(* Logix 5000 AddOnInstructionDefinition export Banner_Q5X_2000_Param_v4; software revision 33.00; part 2 of 3 *)
(* tags used below, declared in another part *)
   Q5X : Banner_Q5X_2000_v4;
   Port_Data : Banner_IOL_Port_v4;
   Port : DINT;
   Local_Control : DINT;
   Command_Being_Processed : BOOL;
   Update_Archive : BOOL;
   Index_Write_Inprocess : INT;
   Index_Write_Control : INT;
   Inprocess_Index : DINT;
(* Banner_Q5X_2000_Param_v4, continued *)

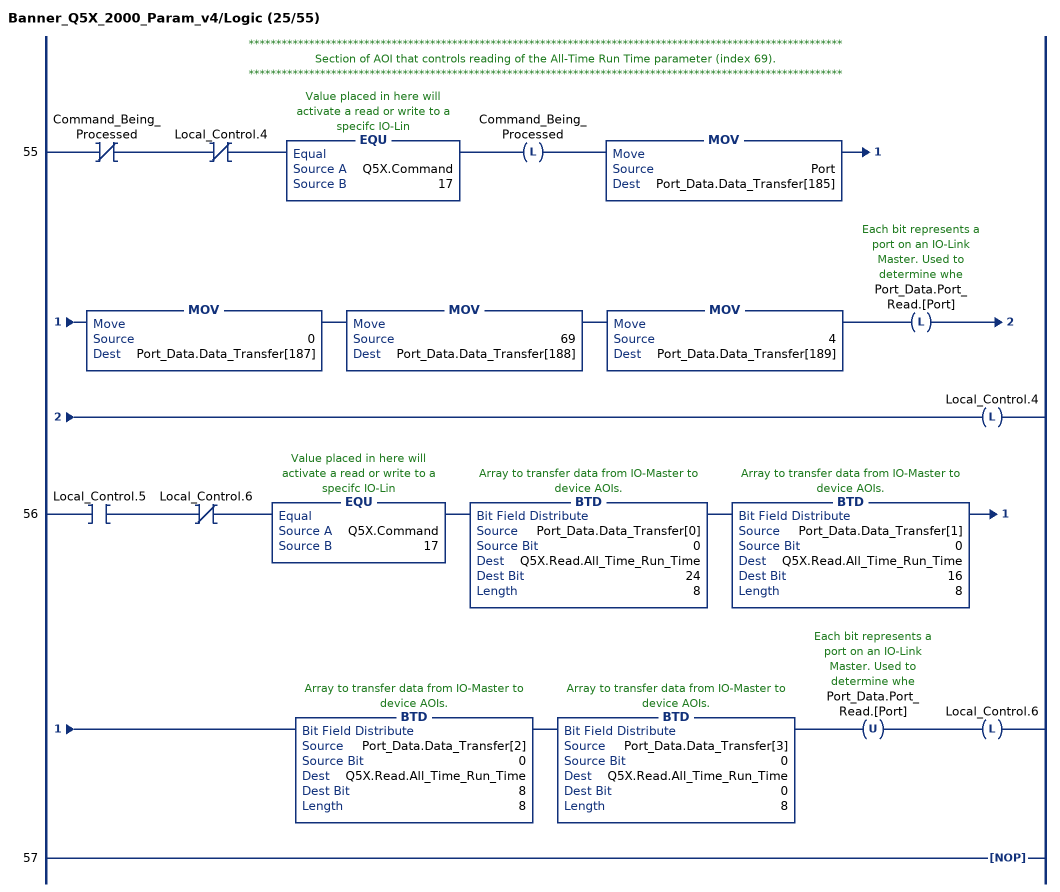
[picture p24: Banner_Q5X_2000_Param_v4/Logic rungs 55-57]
   // ************************************************************************************************************
   // Section of AOI that controls reading of the All-Time Run Time parameter (index 69).
   // ************************************************************************************************************
   55: XIO(Command_Being_Processed)XIO(Local_Control.4)EQU(Q5X.Command,17)OTL(Command_Being_Processed)MOV(Port,Port_Data.Data_Transfer[185])MOV(0,Port_Data.Data_Transfer[187])MOV(69,Port_Data.Data_Transfer[188])MOV(4,Port_Data.Data_Transfer[189])OTL(Port_Data.Port_Read.[Port])OTL(Local_Control.4);
   56: XIC(Local_Control.5)XIO(Local_Control.6)EQU(Q5X.Command,17)BTD(Port_Data.Data_Transfer[0],0,Q5X.Read.All_Time_Run_Time,24,8)BTD(Port_Data.Data_Transfer[1],0,Q5X.Read.All_Time_Run_Time,16,8)BTD(Port_Data.Data_Transfer[2],0,Q5X.Read.All_Time_Run_Time,8,8)BTD(Port_Data.Data_Transfer[3],0,Q5X.Read.All_Time_Run_Time,0,8)OTU(Port_Data.Port_Read.[Port])OTL(Local_Control.6);
   57: NOP();
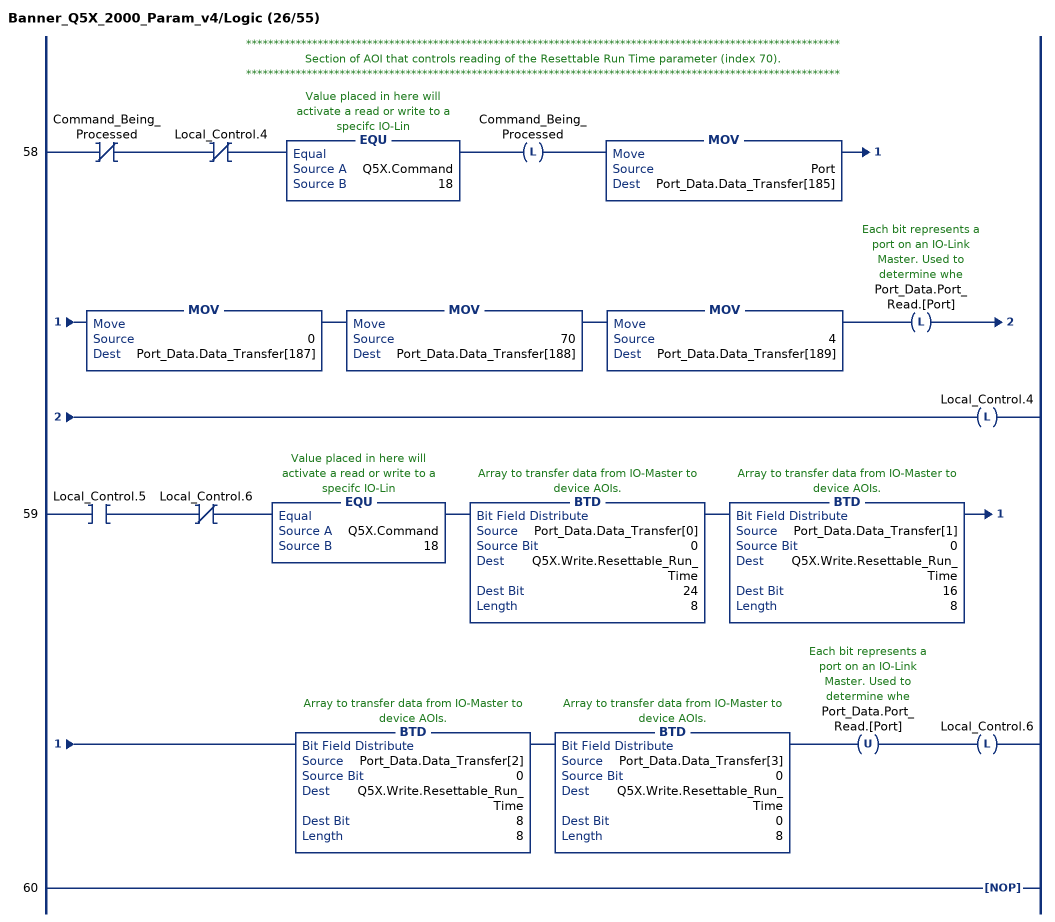
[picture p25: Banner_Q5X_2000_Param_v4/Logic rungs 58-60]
   // ************************************************************************************************************
   // Section of AOI that controls reading of the Resettable Run Time parameter (index 70).
   // ************************************************************************************************************
   58: XIO(Command_Being_Processed)XIO(Local_Control.4)EQU(Q5X.Command,18)OTL(Command_Being_Processed)MOV(Port,Port_Data.Data_Transfer[185])MOV(0,Port_Data.Data_Transfer[187])MOV(70,Port_Data.Data_Transfer[188])MOV(4,Port_Data.Data_Transfer[189])OTL(Port_Data.Port_Read.[Port])OTL(Local_Control.4);
   59: XIC(Local_Control.5)XIO(Local_Control.6)EQU(Q5X.Command,18)BTD(Port_Data.Data_Transfer[0],0,Q5X.Write.Resettable_Run_Time,24,8)BTD(Port_Data.Data_Transfer[1],0,Q5X.Write.Resettable_Run_Time,16,8)BTD(Port_Data.Data_Transfer[2],0,Q5X.Write.Resettable_Run_Time,8,8)BTD(Port_Data.Data_Transfer[3],0,Q5X.Write.Resettable_Run_Time,0,8)OTU(Port_Data.Port_Read.[Port])OTL(Local_Control.6);
   60: NOP();
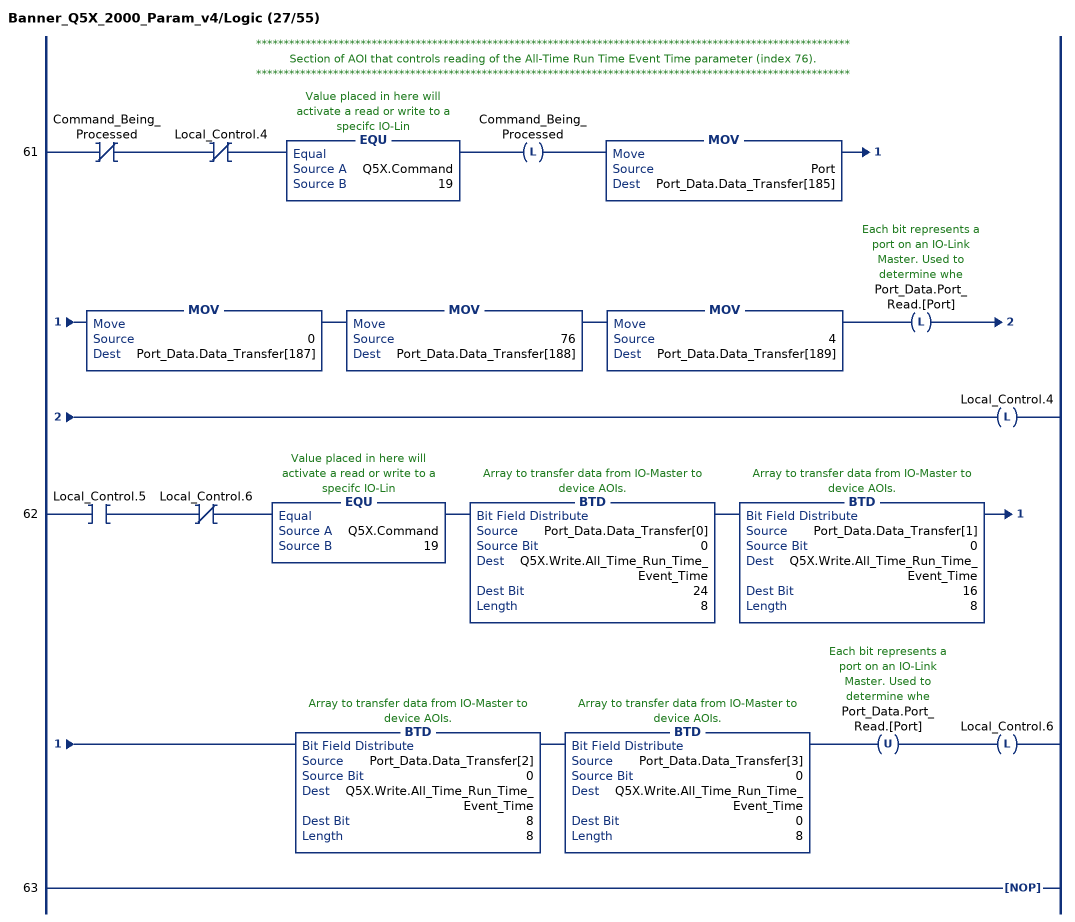
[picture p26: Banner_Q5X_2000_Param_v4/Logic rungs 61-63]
   // ************************************************************************************************************
   // Section of AOI that controls reading of the All-Time Run Time Event Time parameter (index 76).
   // ************************************************************************************************************
   61: XIO(Command_Being_Processed)XIO(Local_Control.4)EQU(Q5X.Command,19)OTL(Command_Being_Processed)MOV(Port,Port_Data.Data_Transfer[185])MOV(0,Port_Data.Data_Transfer[187])MOV(76,Port_Data.Data_Transfer[188])MOV(4,Port_Data.Data_Transfer[189])OTL(Port_Data.Port_Read.[Port])OTL(Local_Control.4);
   62: XIC(Local_Control.5)XIO(Local_Control.6)EQU(Q5X.Command,19)BTD(Port_Data.Data_Transfer[0],0,Q5X.Write.All_Time_Run_Time_Event_Time,24,8)BTD(Port_Data.Data_Transfer[1],0,Q5X.Write.All_Time_Run_Time_Event_Time,16,8)BTD(Port_Data.Data_Transfer[2],0,Q5X.Write.All_Time_Run_Time_Event_Time,8,8)BTD(Port_Data.Data_Transfer[3],0,Q5X.Write.All_Time_Run_Time_Event_Time,0,8)OTU(Port_Data.Port_Read.[Port])OTL(Local_Control.6);
   63: NOP();
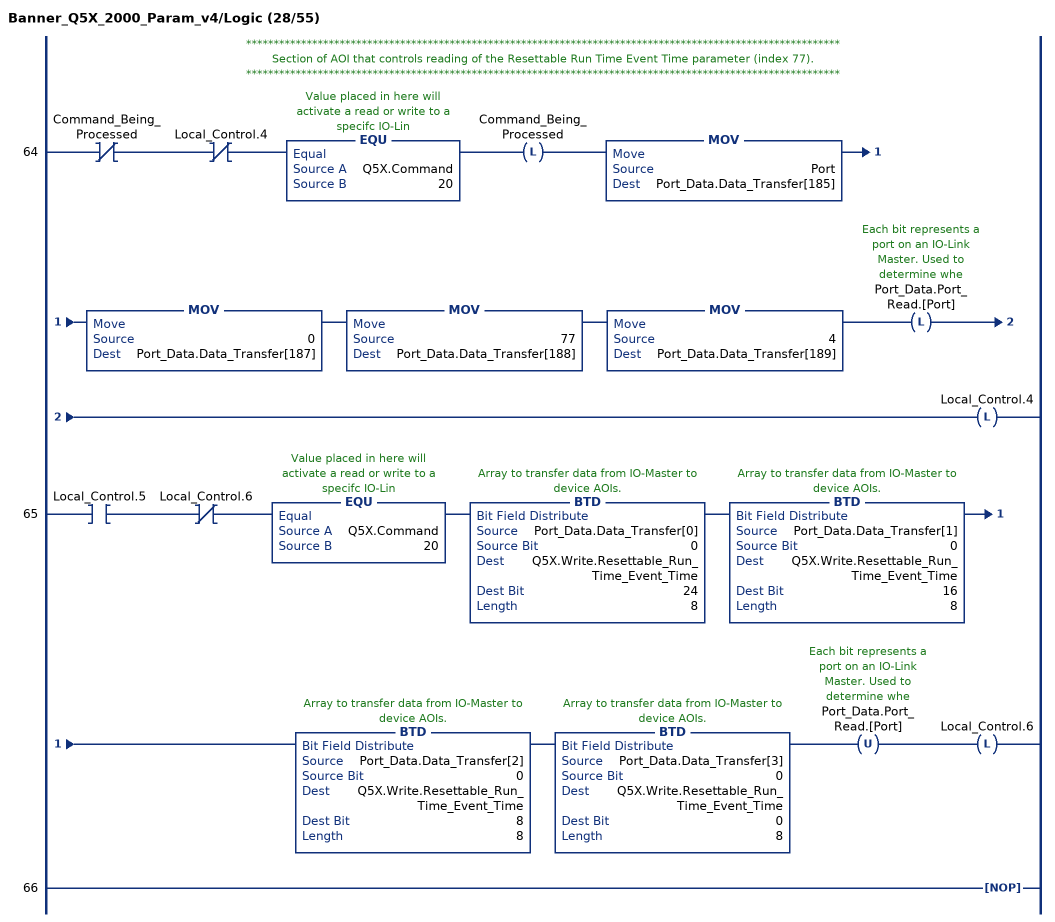
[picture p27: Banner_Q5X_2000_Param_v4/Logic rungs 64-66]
   // ************************************************************************************************************
   // Section of AOI that controls reading of the Resettable Run Time Event Time parameter (index 77).
   // ************************************************************************************************************
   64: XIO(Command_Being_Processed)XIO(Local_Control.4)EQU(Q5X.Command,20)OTL(Command_Being_Processed)MOV(Port,Port_Data.Data_Transfer[185])MOV(0,Port_Data.Data_Transfer[187])MOV(77,Port_Data.Data_Transfer[188])MOV(4,Port_Data.Data_Transfer[189])OTL(Port_Data.Port_Read.[Port])OTL(Local_Control.4);
   65: XIC(Local_Control.5)XIO(Local_Control.6)EQU(Q5X.Command,20)BTD(Port_Data.Data_Transfer[0],0,Q5X.Write.Resettable_Run_Time_Event_Time,24,8)BTD(Port_Data.Data_Transfer[1],0,Q5X.Write.Resettable_Run_Time_Event_Time,16,8)BTD(Port_Data.Data_Transfer[2],0,Q5X.Write.Resettable_Run_Time_Event_Time,8,8)BTD(Port_Data.Data_Transfer[3],0,Q5X.Write.Resettable_Run_Time_Event_Time,0,8)OTU(Port_Data.Port_Read.[Port])OTL(Local_Control.6);
   66: NOP();
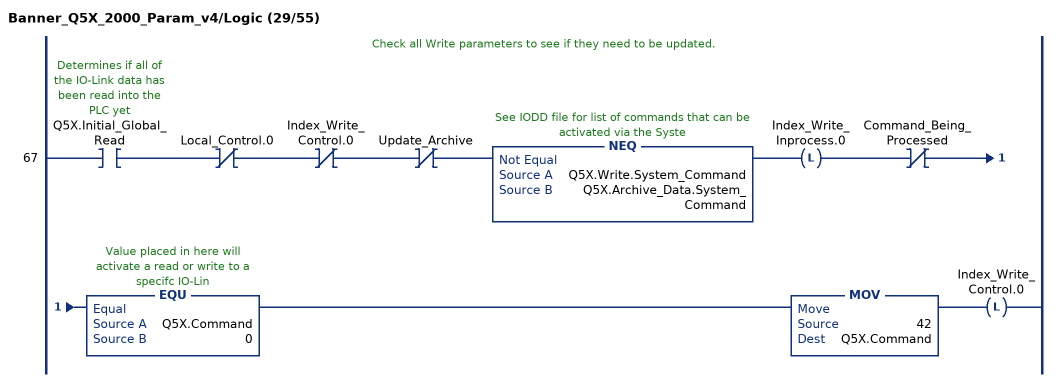
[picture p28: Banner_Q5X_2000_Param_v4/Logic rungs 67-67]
   // Check all Write parameters to see if they need to be updated.
   67: XIC(Q5X.Initial_Global_Read)XIO(Local_Control.0)XIO(Index_Write_Control.0)XIO(Update_Archive)NEQ(Q5X.Write.System_Command,Q5X.Archive_Data.System_Command)OTL(Index_Write_Inprocess.0)XIO(Command_Being_Processed)EQU(Q5X.Command,0)MOV(42,Q5X.Command)OTL(Index_Write_Control.0);
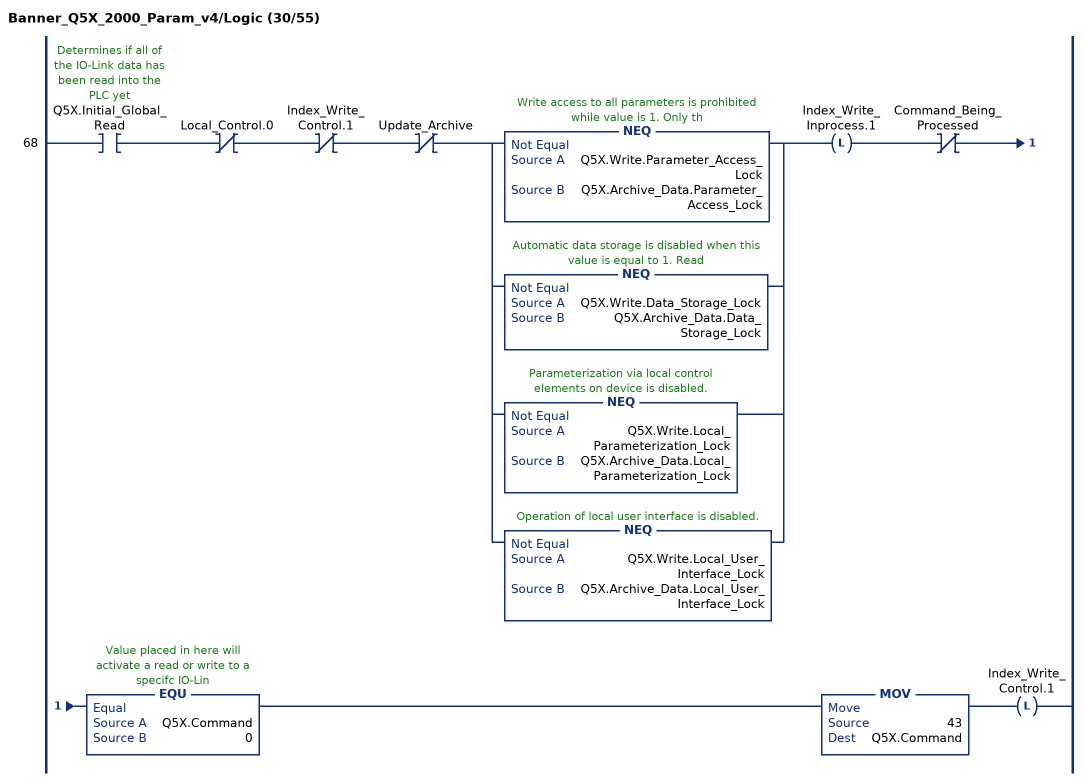
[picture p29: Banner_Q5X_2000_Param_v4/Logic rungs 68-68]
   68: XIC(Q5X.Initial_Global_Read)XIO(Local_Control.0)XIO(Index_Write_Control.1)XIO(Update_Archive)[NEQ(Q5X.Write.Parameter_Access_Lock,Q5X.Archive_Data.Parameter_Access_Lock) ,NEQ(Q5X.Write.Data_Storage_Lock,Q5X.Archive_Data.Data_Storage_Lock) ,NEQ(Q5X.Write.Local_Parameterization_Lock,Q5X.Archive_Data.Local_Parameterization_Lock) ,NEQ(Q5X.Write.Local_User_Interface_Lock,Q5X.Archive_Data.Local_User_Interface_Lock) ]OTL(Index_Write_Inprocess.1)XIO(Command_Being_Processed)EQU(Q5X.Command,0)MOV(43,Q5X.Command)OTL(Index_Write_Control.1);
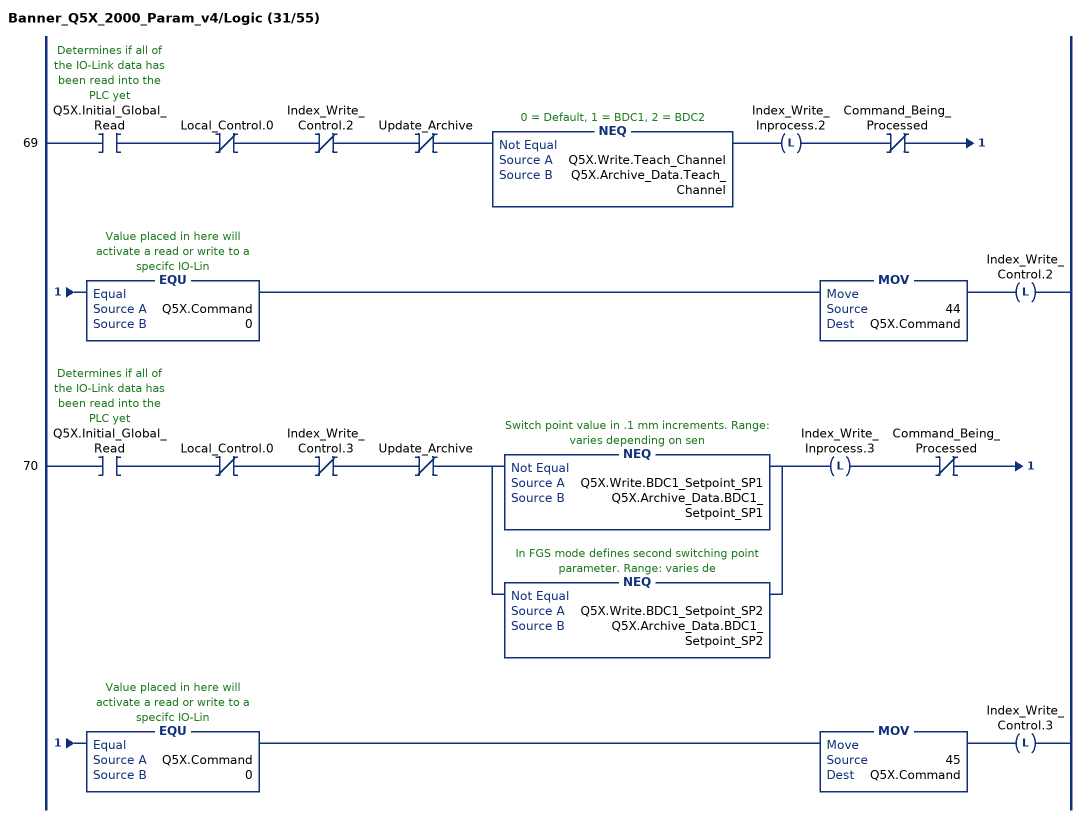
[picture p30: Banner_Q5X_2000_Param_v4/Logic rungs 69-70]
   69: XIC(Q5X.Initial_Global_Read)XIO(Local_Control.0)XIO(Index_Write_Control.2)XIO(Update_Archive)NEQ(Q5X.Write.Teach_Channel,Q5X.Archive_Data.Teach_Channel)OTL(Index_Write_Inprocess.2)XIO(Command_Being_Processed)EQU(Q5X.Command,0)MOV(44,Q5X.Command)OTL(Index_Write_Control.2);
   70: XIC(Q5X.Initial_Global_Read)XIO(Local_Control.0)XIO(Index_Write_Control.3)XIO(Update_Archive)[NEQ(Q5X.Write.BDC1_Setpoint_SP1,Q5X.Archive_Data.BDC1_Setpoint_SP1) ,NEQ(Q5X.Write.BDC1_Setpoint_SP2,Q5X.Archive_Data.BDC1_Setpoint_SP2) ]OTL(Index_Write_Inprocess.3)XIO(Command_Being_Processed)EQU(Q5X.Command,0)MOV(45,Q5X.Command)OTL(Index_Write_Control.3);
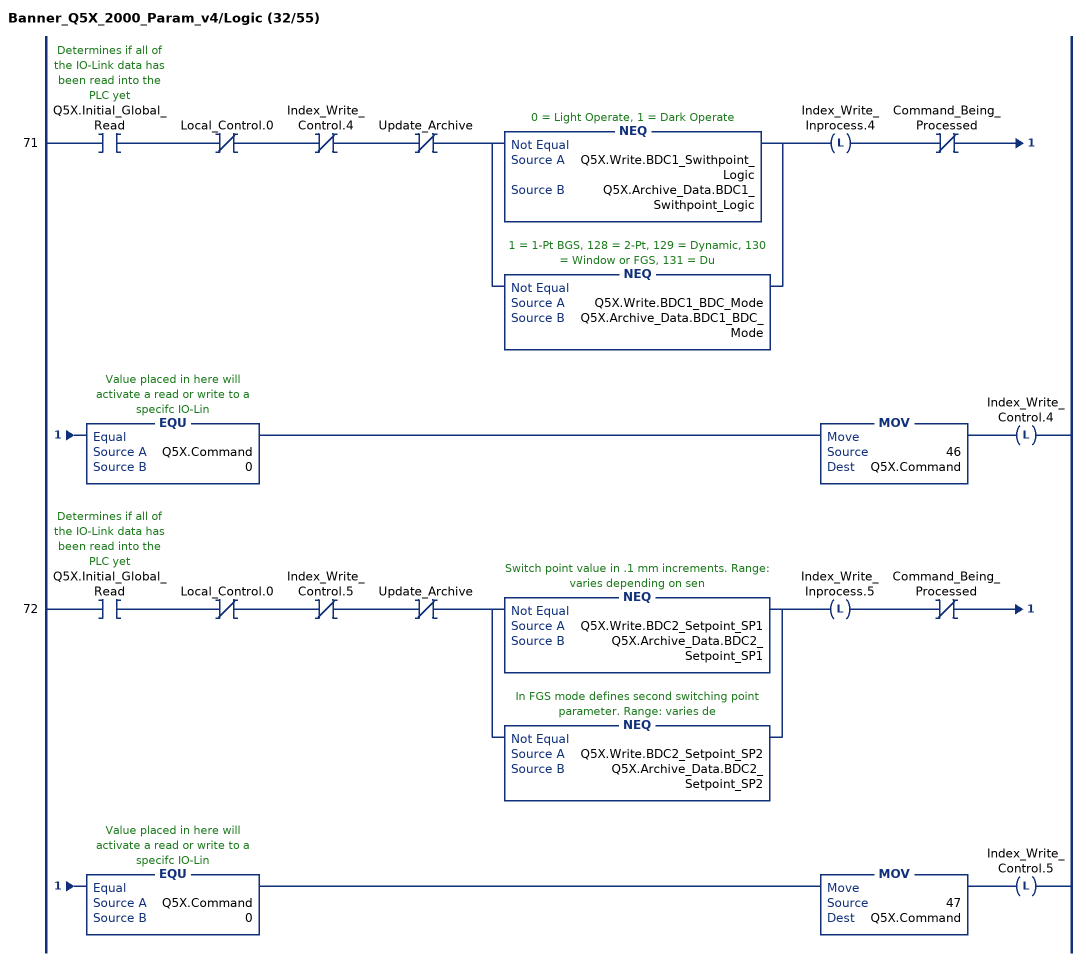
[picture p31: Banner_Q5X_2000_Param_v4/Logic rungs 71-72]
   71: XIC(Q5X.Initial_Global_Read)XIO(Local_Control.0)XIO(Index_Write_Control.4)XIO(Update_Archive)[NEQ(Q5X.Write.BDC1_Swithpoint_Logic,Q5X.Archive_Data.BDC1_Swithpoint_Logic) ,NEQ(Q5X.Write.BDC1_BDC_Mode,Q5X.Archive_Data.BDC1_BDC_Mode) ]OTL(Index_Write_Inprocess.4)XIO(Command_Being_Processed)EQU(Q5X.Command,0)MOV(46,Q5X.Command)OTL(Index_Write_Control.4);
   72: XIC(Q5X.Initial_Global_Read)XIO(Local_Control.0)XIO(Index_Write_Control.5)XIO(Update_Archive)[NEQ(Q5X.Write.BDC2_Setpoint_SP1,Q5X.Archive_Data.BDC2_Setpoint_SP1) ,NEQ(Q5X.Write.BDC2_Setpoint_SP2,Q5X.Archive_Data.BDC2_Setpoint_SP2) ]OTL(Index_Write_Inprocess.5)XIO(Command_Being_Processed)EQU(Q5X.Command,0)MOV(47,Q5X.Command)OTL(Index_Write_Control.5);
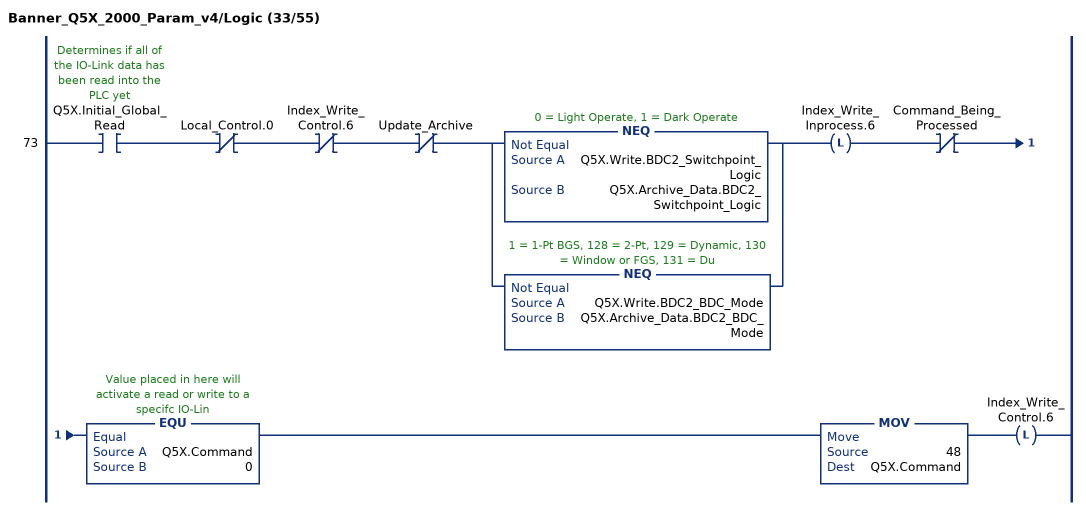
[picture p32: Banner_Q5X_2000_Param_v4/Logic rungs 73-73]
   73: XIC(Q5X.Initial_Global_Read)XIO(Local_Control.0)XIO(Index_Write_Control.6)XIO(Update_Archive)[NEQ(Q5X.Write.BDC2_Switchpoint_Logic,Q5X.Archive_Data.BDC2_Switchpoint_Logic) ,NEQ(Q5X.Write.BDC2_BDC_Mode,Q5X.Archive_Data.BDC2_BDC_Mode) ]OTL(Index_Write_Inprocess.6)XIO(Command_Being_Processed)EQU(Q5X.Command,0)MOV(48,Q5X.Command)OTL(Index_Write_Control.6);
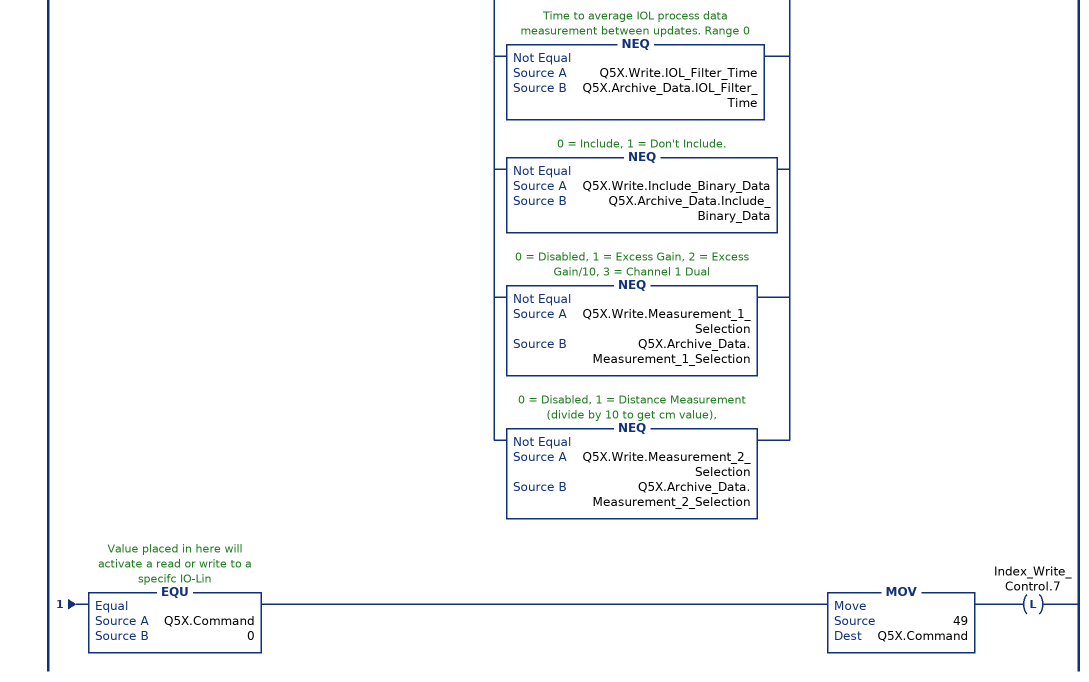
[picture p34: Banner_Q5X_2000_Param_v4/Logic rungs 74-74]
   74: XIC(Q5X.Initial_Global_Read)XIO(Local_Control.0)XIO(Index_Write_Control.7)XIO(Update_Archive)[NEQ(Q5X.Write.Response_Speed,Q5X.Archive_Data.Response_Speed) ,NEQ(Q5X.Write.Gain,Q5X.Archive_Data.Gain) ,NEQ(Q5X.Write.Secondary_Output_Function,Q5X.Archive_Data.Secondary_Output_Function) ,NEQ(Q5X.Write.Zero_Reference_Location,Q5X.Archive_Data.Zero_Reference_Location) ,NEQ(Q5X.Write.Shift_Zero_Reference_After_Teach,Q5X.Archive_Data.Shift_Zero_Reference_After_Teach) ,NEQ(Q5X.Write.Display_Read,Q5X.Archive_Data.Display_Read) ,NEQ(Q5X.Write.Pushbutton_Lockout,Q5X.Archive_Data.Pushbutton_Lockout) ,NEQ(Q5X.Write.Output_Polarity,Q5X.Archive_Data.Output_Polarity) ,NEQ(Q5X.Write.IOL_Filter_Time,Q5X.Archive_Data.IOL_Filter_Time) ,NEQ(Q5X.Write.Include_Binary_Data,Q5X.Archive_Data.Include_Binary_Data) ,NEQ(Q5X.Write.Measurement_1_Selection,Q5X.Archive_Data.Measurement_1_Selection) ,NEQ(Q5X.Write.Measurement_2_Selection,Q5X.Archive_Data.Measurement_2_Selection) ]OTL(Index_Write_Inprocess.7)XIO(Command_Being_Processed)EQU(Q5X.Command,0)MOV(49,Q5X.Command)OTL(Index_Write_Control.7);
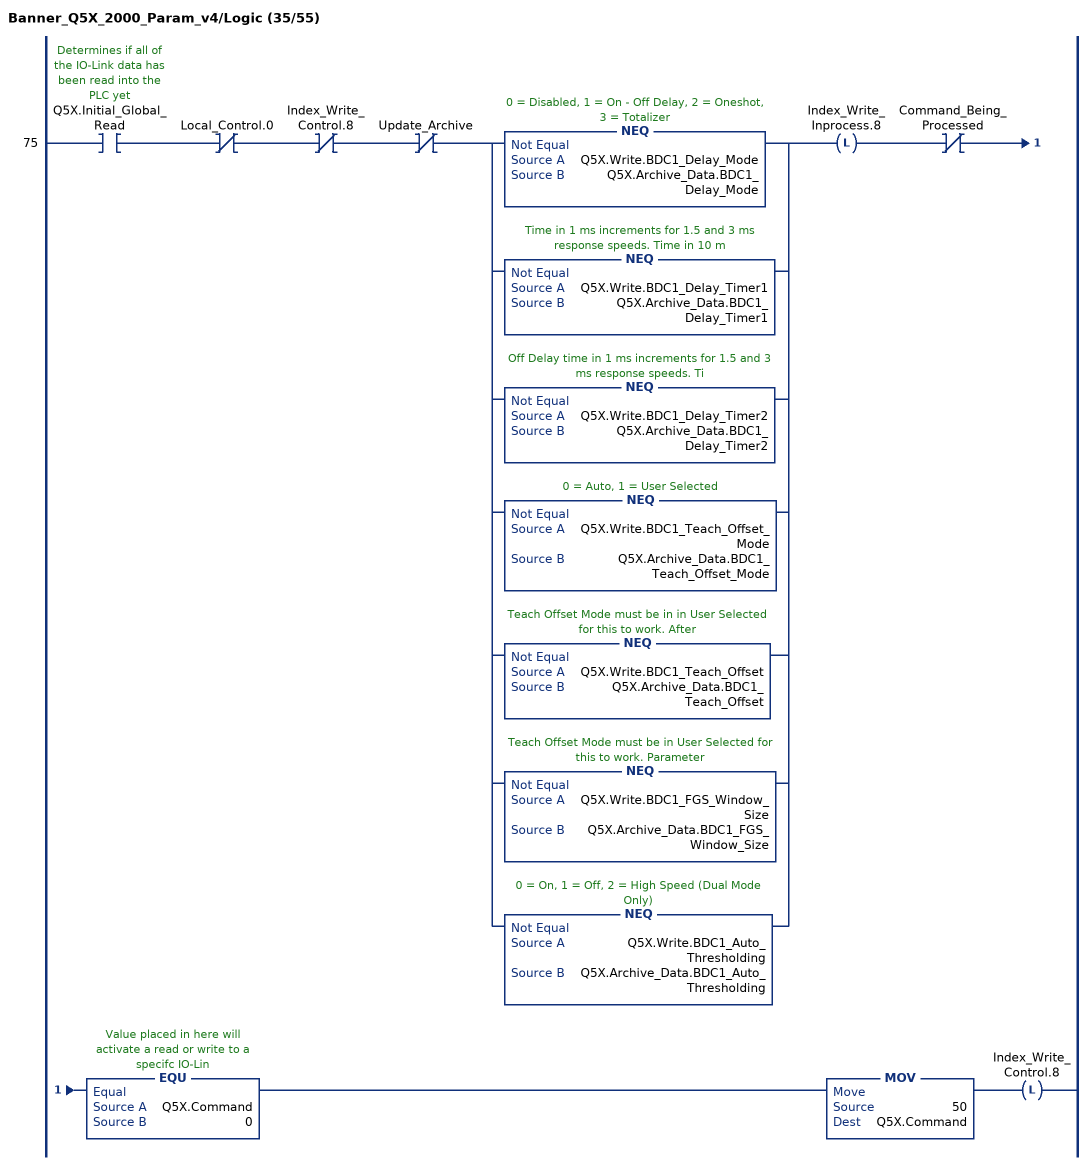
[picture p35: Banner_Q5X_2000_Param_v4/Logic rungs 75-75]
   75: XIC(Q5X.Initial_Global_Read)XIO(Local_Control.0)XIO(Index_Write_Control.8)XIO(Update_Archive)[NEQ(Q5X.Write.BDC1_Delay_Mode,Q5X.Archive_Data.BDC1_Delay_Mode) ,NEQ(Q5X.Write.BDC1_Delay_Timer1,Q5X.Archive_Data.BDC1_Delay_Timer1) ,NEQ(Q5X.Write.BDC1_Delay_Timer2,Q5X.Archive_Data.BDC1_Delay_Timer2) ,NEQ(Q5X.Write.BDC1_Teach_Offset_Mode,Q5X.Archive_Data.BDC1_Teach_Offset_Mode) ,NEQ(Q5X.Write.BDC1_Teach_Offset,Q5X.Archive_Data.BDC1_Teach_Offset) ,NEQ(Q5X.Write.BDC1_FGS_Window_Size,Q5X.Archive_Data.BDC1_FGS_Window_Size) ,NEQ(Q5X.Write.BDC1_Auto_Thresholding,Q5X.Archive_Data.BDC1_Auto_Thresholding) ]OTL(Index_Write_Inprocess.8)XIO(Command_Being_Processed)EQU(Q5X.Command,0)MOV(50,Q5X.Command)OTL(Index_Write_Control.8);
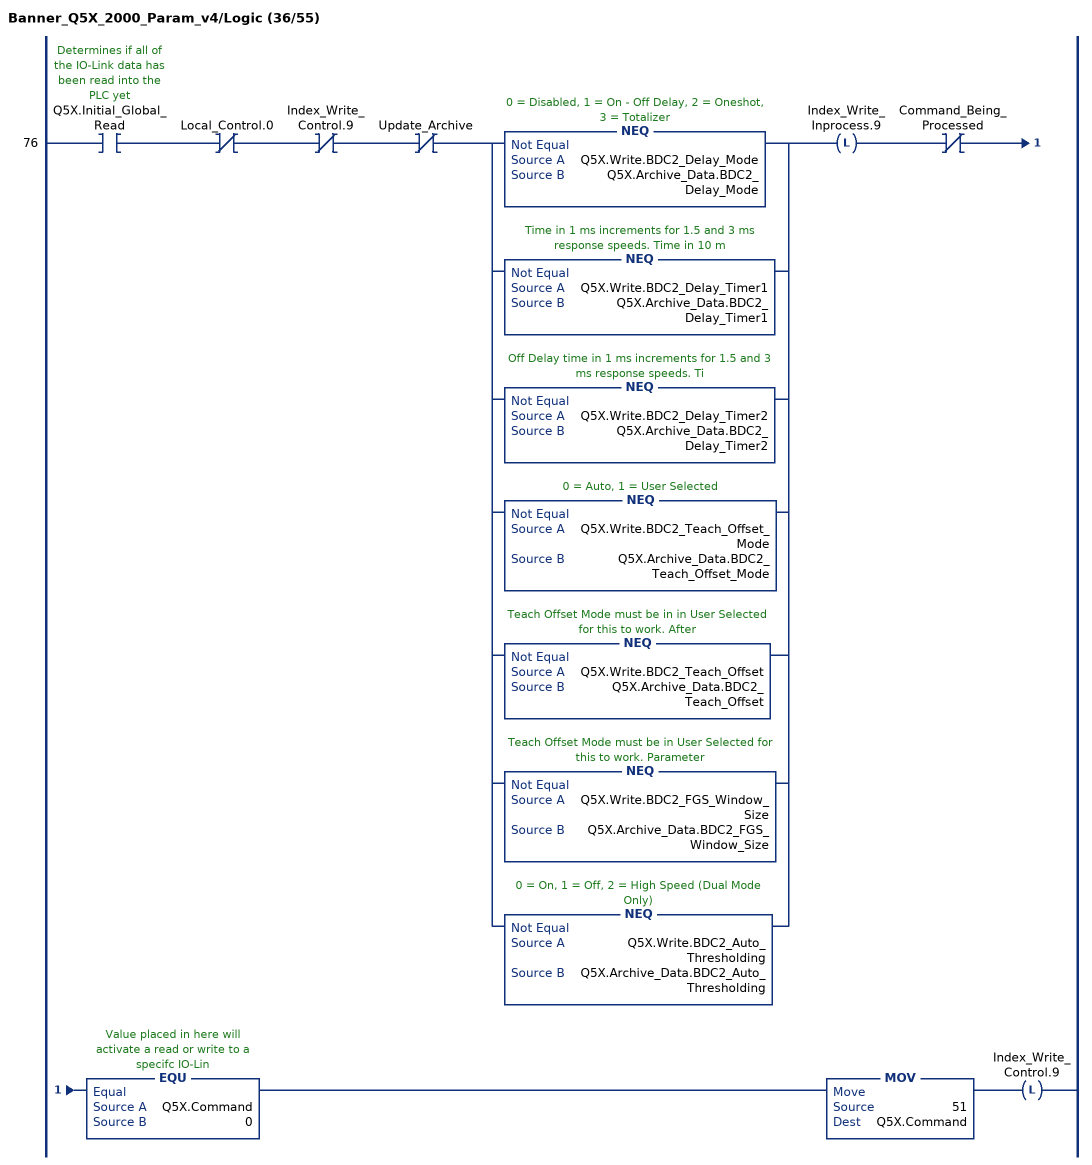
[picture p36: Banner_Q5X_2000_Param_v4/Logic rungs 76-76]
   76: XIC(Q5X.Initial_Global_Read)XIO(Local_Control.0)XIO(Index_Write_Control.9)XIO(Update_Archive)[NEQ(Q5X.Write.BDC2_Delay_Mode,Q5X.Archive_Data.BDC2_Delay_Mode) ,NEQ(Q5X.Write.BDC2_Delay_Timer1,Q5X.Archive_Data.BDC2_Delay_Timer1) ,NEQ(Q5X.Write.BDC2_Delay_Timer2,Q5X.Archive_Data.BDC2_Delay_Timer2) ,NEQ(Q5X.Write.BDC2_Teach_Offset_Mode,Q5X.Archive_Data.BDC2_Teach_Offset_Mode) ,NEQ(Q5X.Write.BDC2_Teach_Offset,Q5X.Archive_Data.BDC2_Teach_Offset) ,NEQ(Q5X.Write.BDC2_FGS_Window_Size,Q5X.Archive_Data.BDC2_FGS_Window_Size) ,NEQ(Q5X.Write.BDC2_Auto_Thresholding,Q5X.Archive_Data.BDC2_Auto_Thresholding) ]OTL(Index_Write_Inprocess.9)XIO(Command_Being_Processed)EQU(Q5X.Command,0)MOV(51,Q5X.Command)OTL(Index_Write_Control.9);
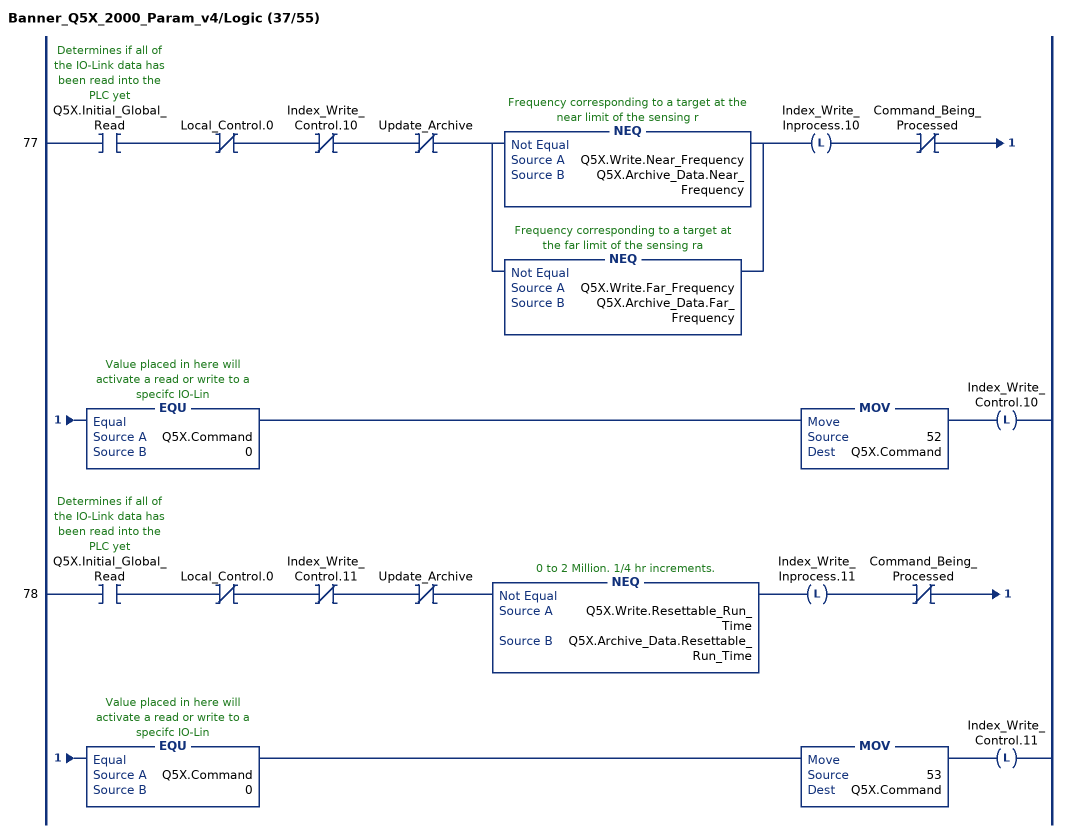
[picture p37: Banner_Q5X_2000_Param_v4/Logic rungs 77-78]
   77: XIC(Q5X.Initial_Global_Read)XIO(Local_Control.0)XIO(Index_Write_Control.10)XIO(Update_Archive)[NEQ(Q5X.Write.Near_Frequency,Q5X.Archive_Data.Near_Frequency) ,NEQ(Q5X.Write.Far_Frequency,Q5X.Archive_Data.Far_Frequency) ]OTL(Index_Write_Inprocess.10)XIO(Command_Being_Processed)EQU(Q5X.Command,0)MOV(52,Q5X.Command)OTL(Index_Write_Control.10);
   78: XIC(Q5X.Initial_Global_Read)XIO(Local_Control.0)XIO(Index_Write_Control.11)XIO(Update_Archive)NEQ(Q5X.Write.Resettable_Run_Time,Q5X.Archive_Data.Resettable_Run_Time)OTL(Index_Write_Inprocess.11)XIO(Command_Being_Processed)EQU(Q5X.Command,0)MOV(53,Q5X.Command)OTL(Index_Write_Control.11);
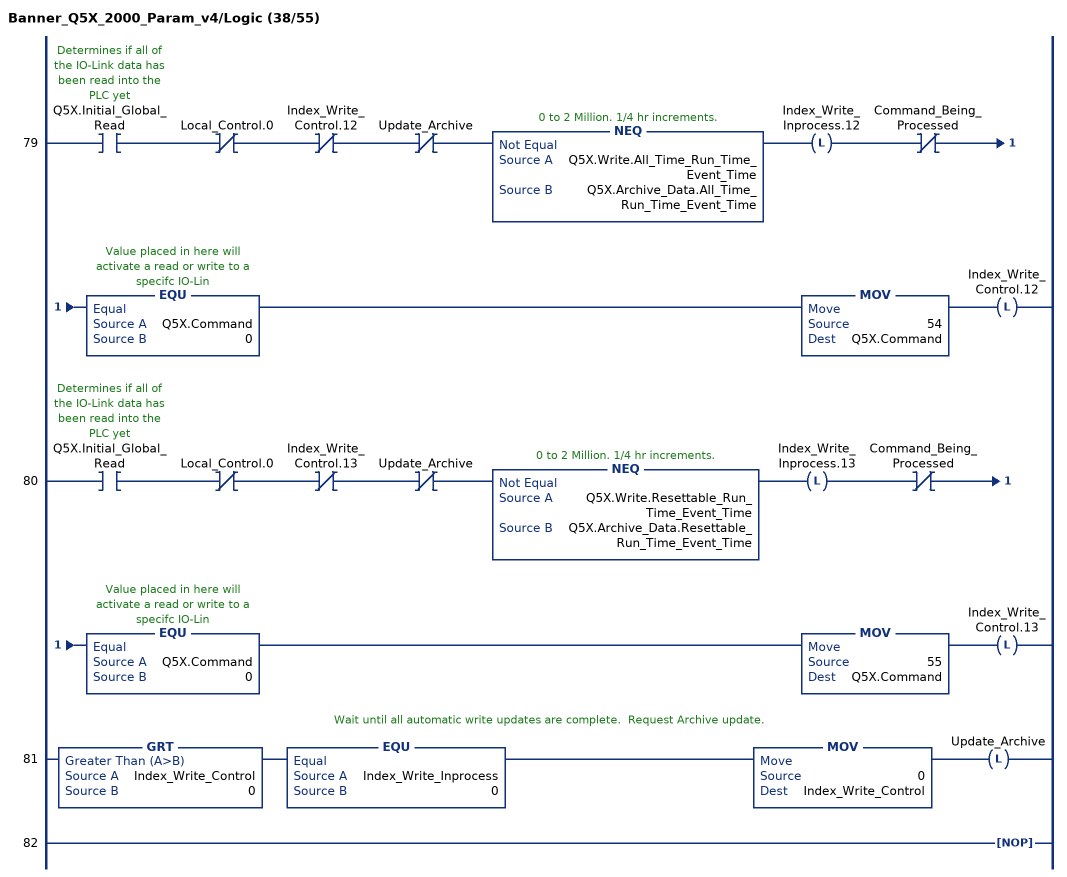
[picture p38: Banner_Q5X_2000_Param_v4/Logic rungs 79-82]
   79: XIC(Q5X.Initial_Global_Read)XIO(Local_Control.0)XIO(Index_Write_Control.12)XIO(Update_Archive)NEQ(Q5X.Write.All_Time_Run_Time_Event_Time,Q5X.Archive_Data.All_Time_Run_Time_Event_Time)OTL(Index_Write_Inprocess.12)XIO(Command_Being_Processed)EQU(Q5X.Command,0)MOV(54,Q5X.Command)OTL(Index_Write_Control.12);
   80: XIC(Q5X.Initial_Global_Read)XIO(Local_Control.0)XIO(Index_Write_Control.13)XIO(Update_Archive)NEQ(Q5X.Write.Resettable_Run_Time_Event_Time,Q5X.Archive_Data.Resettable_Run_Time_Event_Time)OTL(Index_Write_Inprocess.13)XIO(Command_Being_Processed)EQU(Q5X.Command,0)MOV(55,Q5X.Command)OTL(Index_Write_Control.13);
   // Wait until all automatic write updates are complete.  Request Archive update.
   81: GRT(Index_Write_Control,0)EQU(Index_Write_Inprocess,0)MOV(0,Index_Write_Control)OTL(Update_Archive);
   82: NOP();
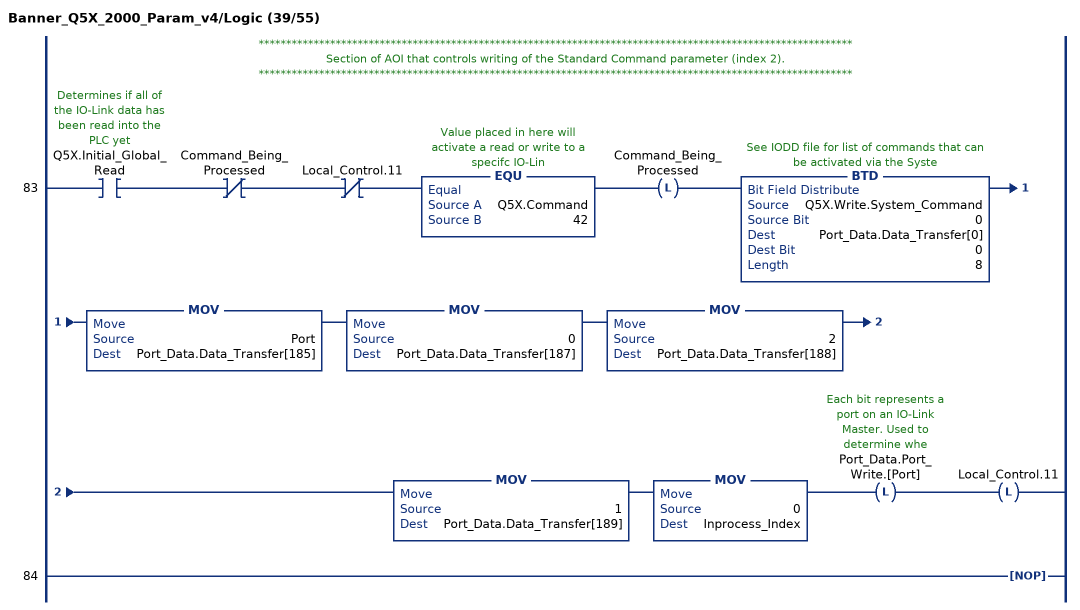
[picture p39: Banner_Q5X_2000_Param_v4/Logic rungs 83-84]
   // ************************************************************************************************************
   // Section of AOI that controls writing of the Standard Command parameter (index 2).
   // ************************************************************************************************************
   83: XIC(Q5X.Initial_Global_Read)XIO(Command_Being_Processed)XIO(Local_Control.11)EQU(Q5X.Command,42)OTL(Command_Being_Processed)BTD(Q5X.Write.System_Command,0,Port_Data.Data_Transfer[0],0,8)MOV(Port,Port_Data.Data_Transfer[185])MOV(0,Port_Data.Data_Transfer[187])MOV(2,Port_Data.Data_Transfer[188])MOV(1,Port_Data.Data_Transfer[189])MOV(0,Inprocess_Index)OTL(Port_Data.Port_Write.[Port])OTL(Local_Control.11);
   84: NOP();
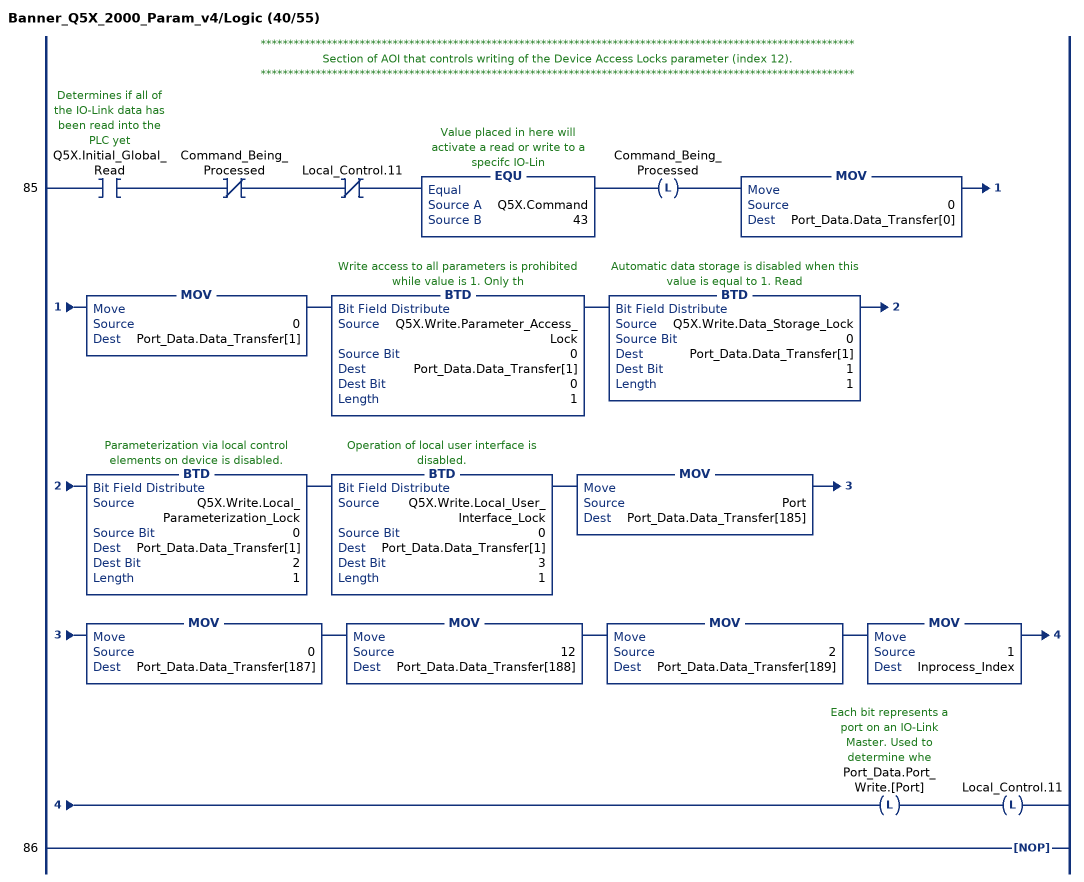
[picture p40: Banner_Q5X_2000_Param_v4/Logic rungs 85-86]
   // ************************************************************************************************************
   // Section of AOI that controls writing of the Device Access Locks parameter (index 12).
   // ************************************************************************************************************
   85: XIC(Q5X.Initial_Global_Read)XIO(Command_Being_Processed)XIO(Local_Control.11)EQU(Q5X.Command,43)OTL(Command_Being_Processed)MOV(0,Port_Data.Data_Transfer[0])MOV(0,Port_Data.Data_Transfer[1])BTD(Q5X.Write.Parameter_Access_Lock,0,Port_Data.Data_Transfer[1],0,1)BTD(Q5X.Write.Data_Storage_Lock,0,Port_Data.Data_Transfer[1],1,1)BTD(Q5X.Write.Local_Parameterization_Lock,0,Port_Data.Data_Transfer[1],2,1)BTD(Q5X.Write.Local_User_Interface_Lock,0,Port_Data.Data_Transfer[1],3,1)MOV(Port,Port_Data.Data_Transfer[185])MOV(0,Port_Data.Data_Transfer[187])MOV(12,Port_Data.Data_Transfer[188])MOV(2,Port_Data.Data_Transfer[189])MOV(1,Inprocess_Index)OTL(Port_Data.Port_Write.[Port])OTL(Local_Control.11);
   86: NOP();
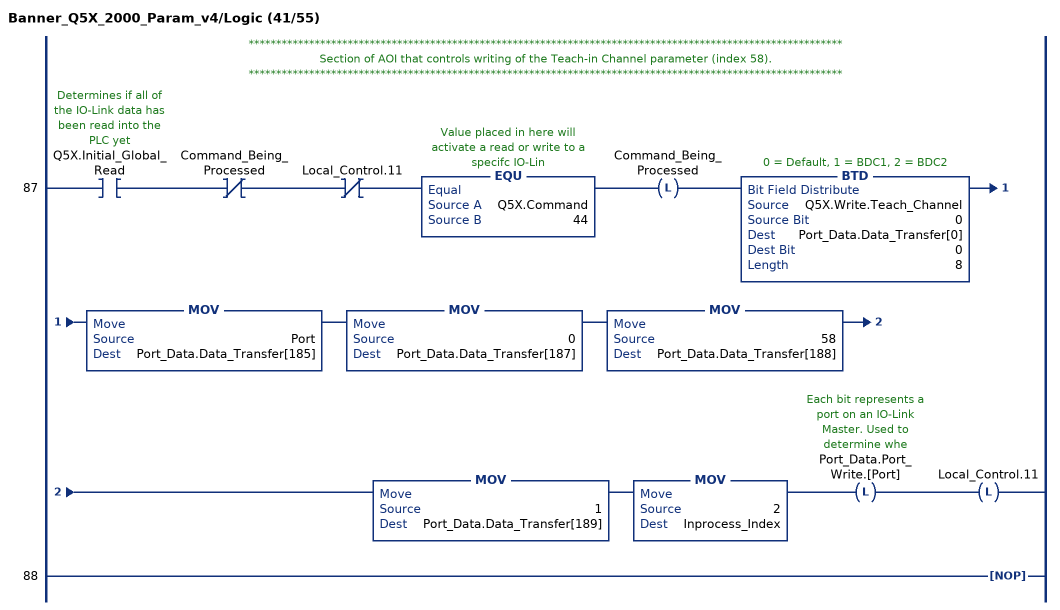
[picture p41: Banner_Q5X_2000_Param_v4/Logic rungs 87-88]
   // ************************************************************************************************************
   // Section of AOI that controls writing of the Teach-in Channel parameter (index 58).
   // ************************************************************************************************************
   87: XIC(Q5X.Initial_Global_Read)XIO(Command_Being_Processed)XIO(Local_Control.11)EQU(Q5X.Command,44)OTL(Command_Being_Processed)BTD(Q5X.Write.Teach_Channel,0,Port_Data.Data_Transfer[0],0,8)MOV(Port,Port_Data.Data_Transfer[185])MOV(0,Port_Data.Data_Transfer[187])MOV(58,Port_Data.Data_Transfer[188])MOV(1,Port_Data.Data_Transfer[189])MOV(2,Inprocess_Index)OTL(Port_Data.Port_Write.[Port])OTL(Local_Control.11);
   88: NOP();
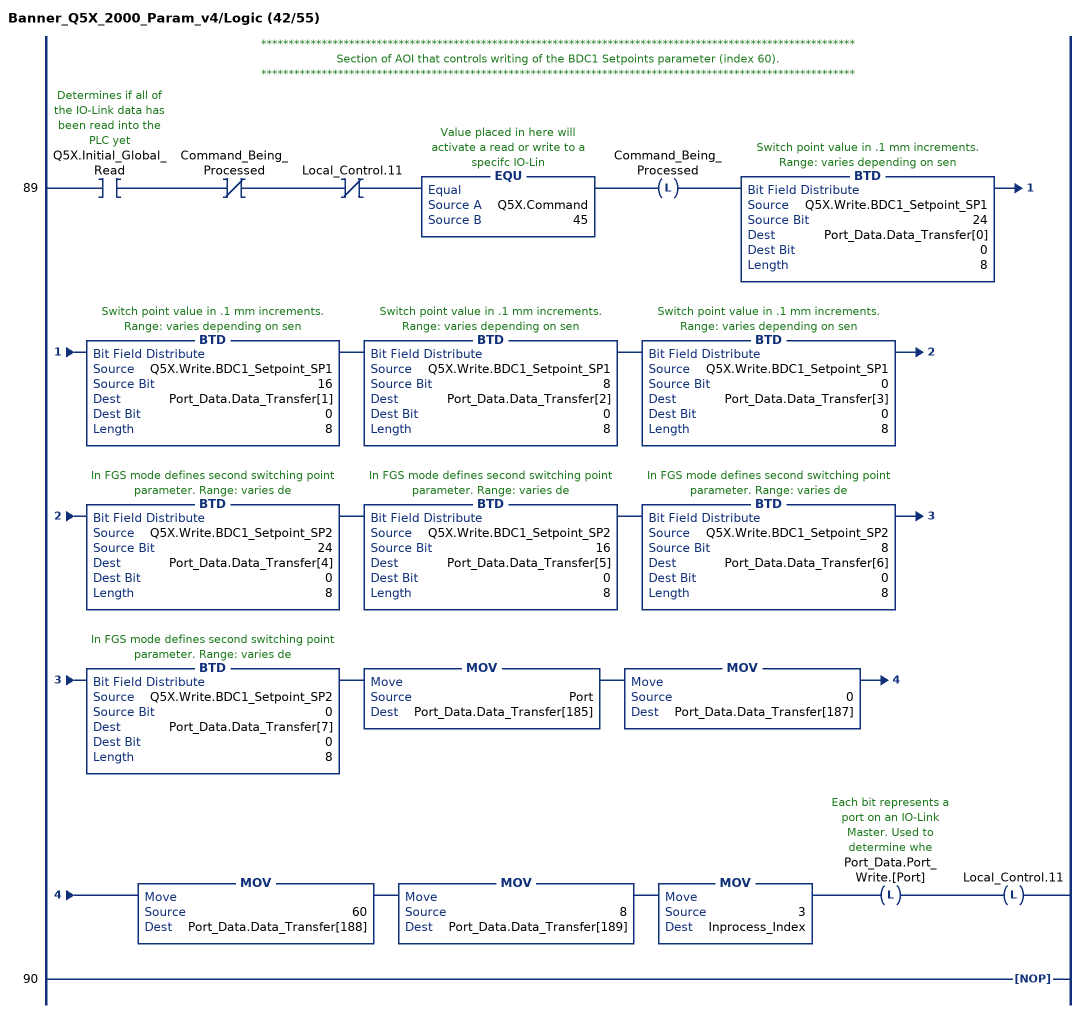
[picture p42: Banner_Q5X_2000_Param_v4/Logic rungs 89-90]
   // ************************************************************************************************************
   // Section of AOI that controls writing of the BDC1 Setpoints parameter (index 60).
   // ************************************************************************************************************
   89: XIC(Q5X.Initial_Global_Read)XIO(Command_Being_Processed)XIO(Local_Control.11)EQU(Q5X.Command,45)OTL(Command_Being_Processed)BTD(Q5X.Write.BDC1_Setpoint_SP1,24,Port_Data.Data_Transfer[0],0,8)BTD(Q5X.Write.BDC1_Setpoint_SP1,16,Port_Data.Data_Transfer[1],0,8)BTD(Q5X.Write.BDC1_Setpoint_SP1,8,Port_Data.Data_Transfer[2],0,8)BTD(Q5X.Write.BDC1_Setpoint_SP1,0,Port_Data.Data_Transfer[3],0,8)BTD(Q5X.Write.BDC1_Setpoint_SP2,24,Port_Data.Data_Transfer[4],0,8)BTD(Q5X.Write.BDC1_Setpoint_SP2,16,Port_Data.Data_Transfer[5],0,8)BTD(Q5X.Write.BDC1_Setpoint_SP2,8,Port_Data.Data_Transfer[6],0,8)BTD(Q5X.Write.BDC1_Setpoint_SP2,0,Port_Data.Data_Transfer[7],0,8)MOV(Port,Port_Data.Data_Transfer[185])MOV(0,Port_Data.Data_Transfer[187])MOV(60,Port_Data.Data_Transfer[188])MOV(8,Port_Data.Data_Transfer[189])MOV(3,Inprocess_Index)OTL(Port_Data.Port_Write.[Port])OTL(Local_Control.11);
   90: NOP();
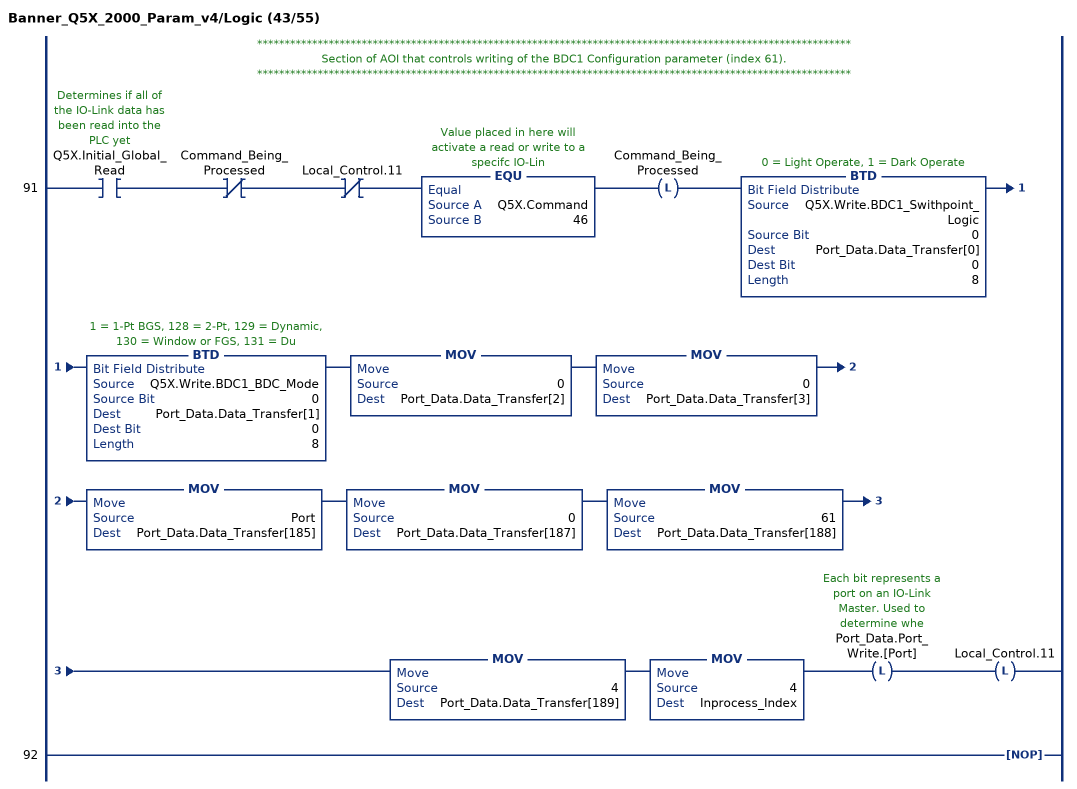
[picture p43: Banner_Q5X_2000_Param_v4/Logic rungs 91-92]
   // ************************************************************************************************************
   // Section of AOI that controls writing of the BDC1 Configuration parameter (index 61).
   // ************************************************************************************************************
   91: XIC(Q5X.Initial_Global_Read)XIO(Command_Being_Processed)XIO(Local_Control.11)EQU(Q5X.Command,46)OTL(Command_Being_Processed)BTD(Q5X.Write.BDC1_Swithpoint_Logic,0,Port_Data.Data_Transfer[0],0,8)BTD(Q5X.Write.BDC1_BDC_Mode,0,Port_Data.Data_Transfer[1],0,8)MOV(0,Port_Data.Data_Transfer[2])MOV(0,Port_Data.Data_Transfer[3])MOV(Port,Port_Data.Data_Transfer[185])MOV(0,Port_Data.Data_Transfer[187])MOV(61,Port_Data.Data_Transfer[188])MOV(4,Port_Data.Data_Transfer[189])MOV(4,Inprocess_Index)OTL(Port_Data.Port_Write.[Port])OTL(Local_Control.11);
   92: NOP();
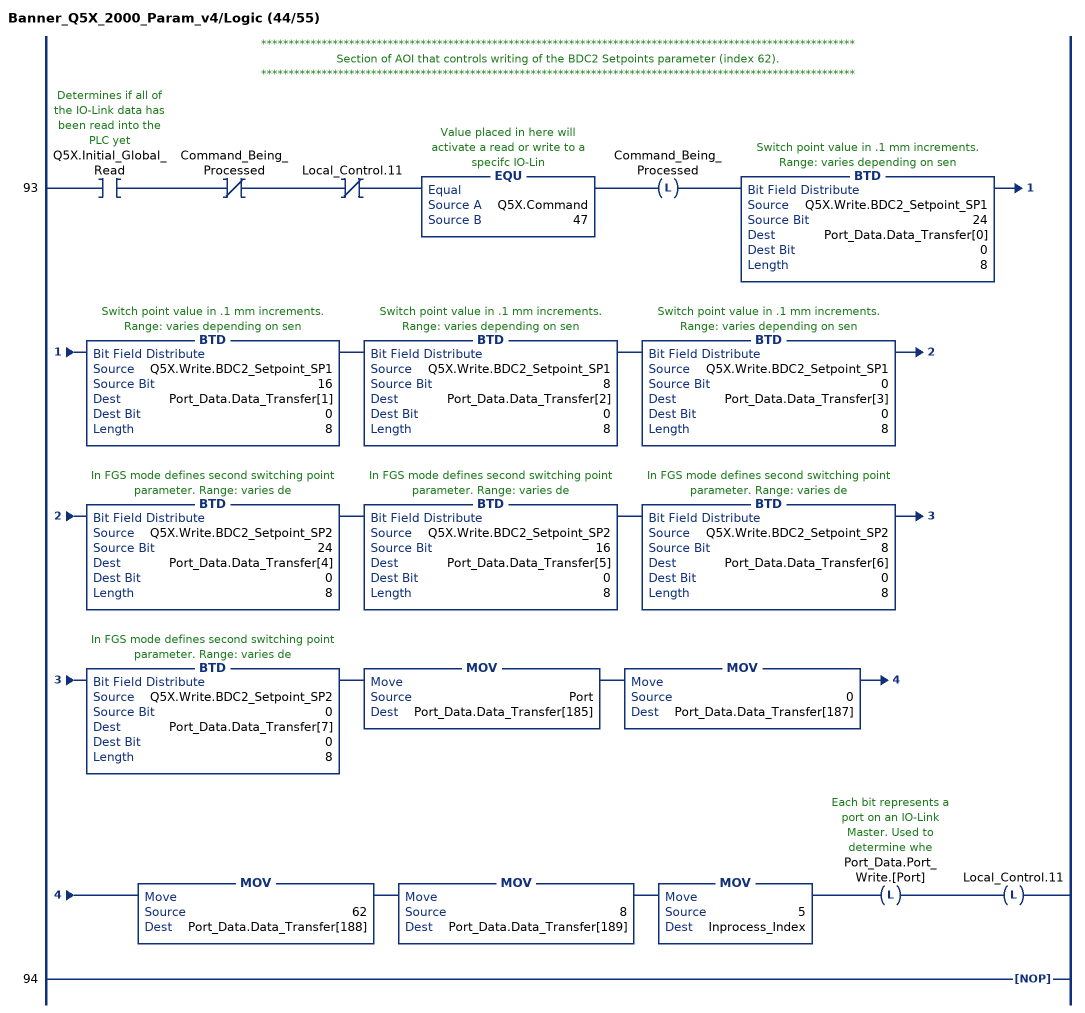
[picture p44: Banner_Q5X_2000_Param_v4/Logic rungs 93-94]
   // ************************************************************************************************************
   // Section of AOI that controls writing of the BDC2 Setpoints parameter (index 62).
   // ************************************************************************************************************
   93: XIC(Q5X.Initial_Global_Read)XIO(Command_Being_Processed)XIO(Local_Control.11)EQU(Q5X.Command,47)OTL(Command_Being_Processed)BTD(Q5X.Write.BDC2_Setpoint_SP1,24,Port_Data.Data_Transfer[0],0,8)BTD(Q5X.Write.BDC2_Setpoint_SP1,16,Port_Data.Data_Transfer[1],0,8)BTD(Q5X.Write.BDC2_Setpoint_SP1,8,Port_Data.Data_Transfer[2],0,8)BTD(Q5X.Write.BDC2_Setpoint_SP1,0,Port_Data.Data_Transfer[3],0,8)BTD(Q5X.Write.BDC2_Setpoint_SP2,24,Port_Data.Data_Transfer[4],0,8)BTD(Q5X.Write.BDC2_Setpoint_SP2,16,Port_Data.Data_Transfer[5],0,8)BTD(Q5X.Write.BDC2_Setpoint_SP2,8,Port_Data.Data_Transfer[6],0,8)BTD(Q5X.Write.BDC2_Setpoint_SP2,0,Port_Data.Data_Transfer[7],0,8)MOV(Port,Port_Data.Data_Transfer[185])MOV(0,Port_Data.Data_Transfer[187])MOV(62,Port_Data.Data_Transfer[188])MOV(8,Port_Data.Data_Transfer[189])MOV(5,Inprocess_Index)OTL(Port_Data.Port_Write.[Port])OTL(Local_Control.11);
   94: NOP();
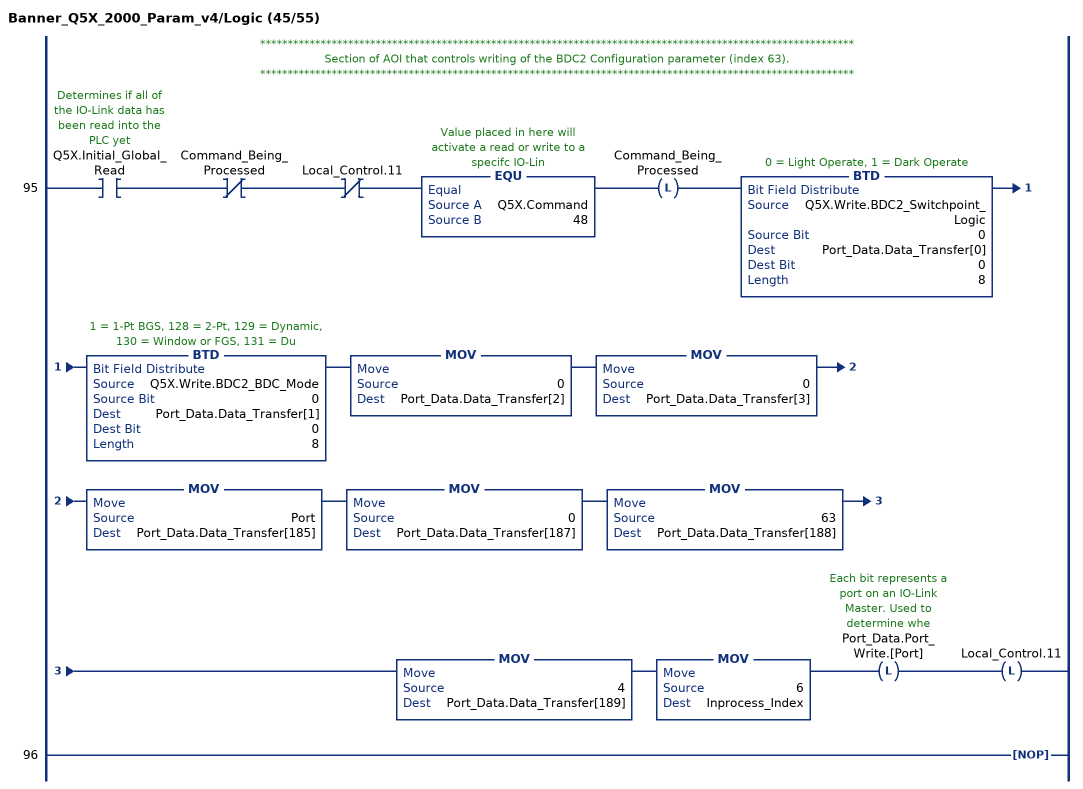
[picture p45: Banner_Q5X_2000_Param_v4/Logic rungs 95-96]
   // ************************************************************************************************************
   // Section of AOI that controls writing of the BDC2 Configuration parameter (index 63).
   // ************************************************************************************************************
   95: XIC(Q5X.Initial_Global_Read)XIO(Command_Being_Processed)XIO(Local_Control.11)EQU(Q5X.Command,48)OTL(Command_Being_Processed)BTD(Q5X.Write.BDC2_Switchpoint_Logic,0,Port_Data.Data_Transfer[0],0,8)BTD(Q5X.Write.BDC2_BDC_Mode,0,Port_Data.Data_Transfer[1],0,8)MOV(0,Port_Data.Data_Transfer[2])MOV(0,Port_Data.Data_Transfer[3])MOV(Port,Port_Data.Data_Transfer[185])MOV(0,Port_Data.Data_Transfer[187])MOV(63,Port_Data.Data_Transfer[188])MOV(4,Port_Data.Data_Transfer[189])MOV(6,Inprocess_Index)OTL(Port_Data.Port_Write.[Port])OTL(Local_Control.11);
   96: NOP();
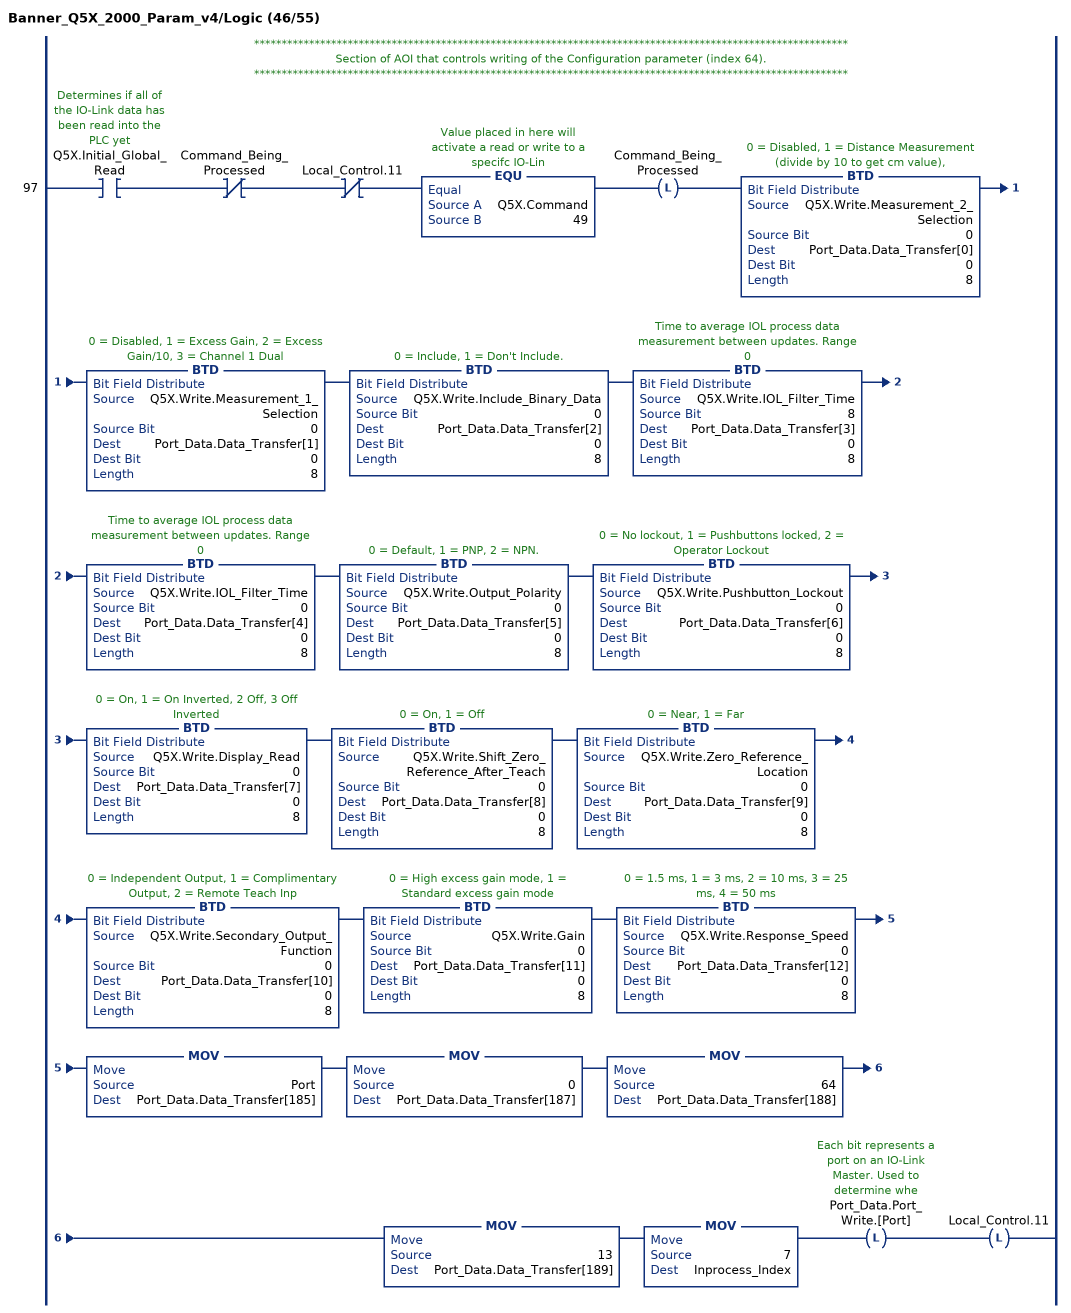
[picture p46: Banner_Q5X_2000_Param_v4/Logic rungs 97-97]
   // ************************************************************************************************************
   // Section of AOI that controls writing of the Configuration parameter (index 64).
   // ************************************************************************************************************
   97: XIC(Q5X.Initial_Global_Read)XIO(Command_Being_Processed)XIO(Local_Control.11)EQU(Q5X.Command,49)OTL(Command_Being_Processed)BTD(Q5X.Write.Measurement_2_Selection,0,Port_Data.Data_Transfer[0],0,8)BTD(Q5X.Write.Measurement_1_Selection,0,Port_Data.Data_Transfer[1],0,8)BTD(Q5X.Write.Include_Binary_Data,0,Port_Data.Data_Transfer[2],0,8)BTD(Q5X.Write.IOL_Filter_Time,8,Port_Data.Data_Transfer[3],0,8)BTD(Q5X.Write.IOL_Filter_Time,0,Port_Data.Data_Transfer[4],0,8)BTD(Q5X.Write.Output_Polarity,0,Port_Data.Data_Transfer[5],0,8)BTD(Q5X.Write.Pushbutton_Lockout,0,Port_Data.Data_Transfer[6],0,8)BTD(Q5X.Write.Display_Read,0,Port_Data.Data_Transfer[7],0,8)BTD(Q5X.Write.Shift_Zero_Reference_After_Teach,0,Port_Data.Data_Transfer[8],0,8)BTD(Q5X.Write.Zero_Reference_Location,0,Port_Data.Data_Transfer[9],0,8)BTD(Q5X.Write.Secondary_Output_Function,0,Port_Data.Data_Transfer[10],0,8)BTD(Q5X.Write.Gain,0,Port_Data.Data_Transfer[11],0,8)BTD(Q5X.Write.Response_Speed,0,Port_Data.Data_Transfer[12],0,8)MOV(Port,Port_Data.Data_Transfer[185])MOV(0,Port_Data.Data_Transfer[187])MOV(64,Port_Data.Data_Transfer[188])MOV(13,Port_Data.Data_Transfer[189])MOV(7,Inprocess_Index)OTL(Port_Data.Port_Write.[Port])OTL(Local_Control.11);
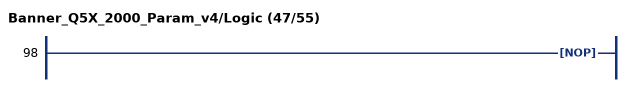
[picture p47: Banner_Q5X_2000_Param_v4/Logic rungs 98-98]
   98: NOP();
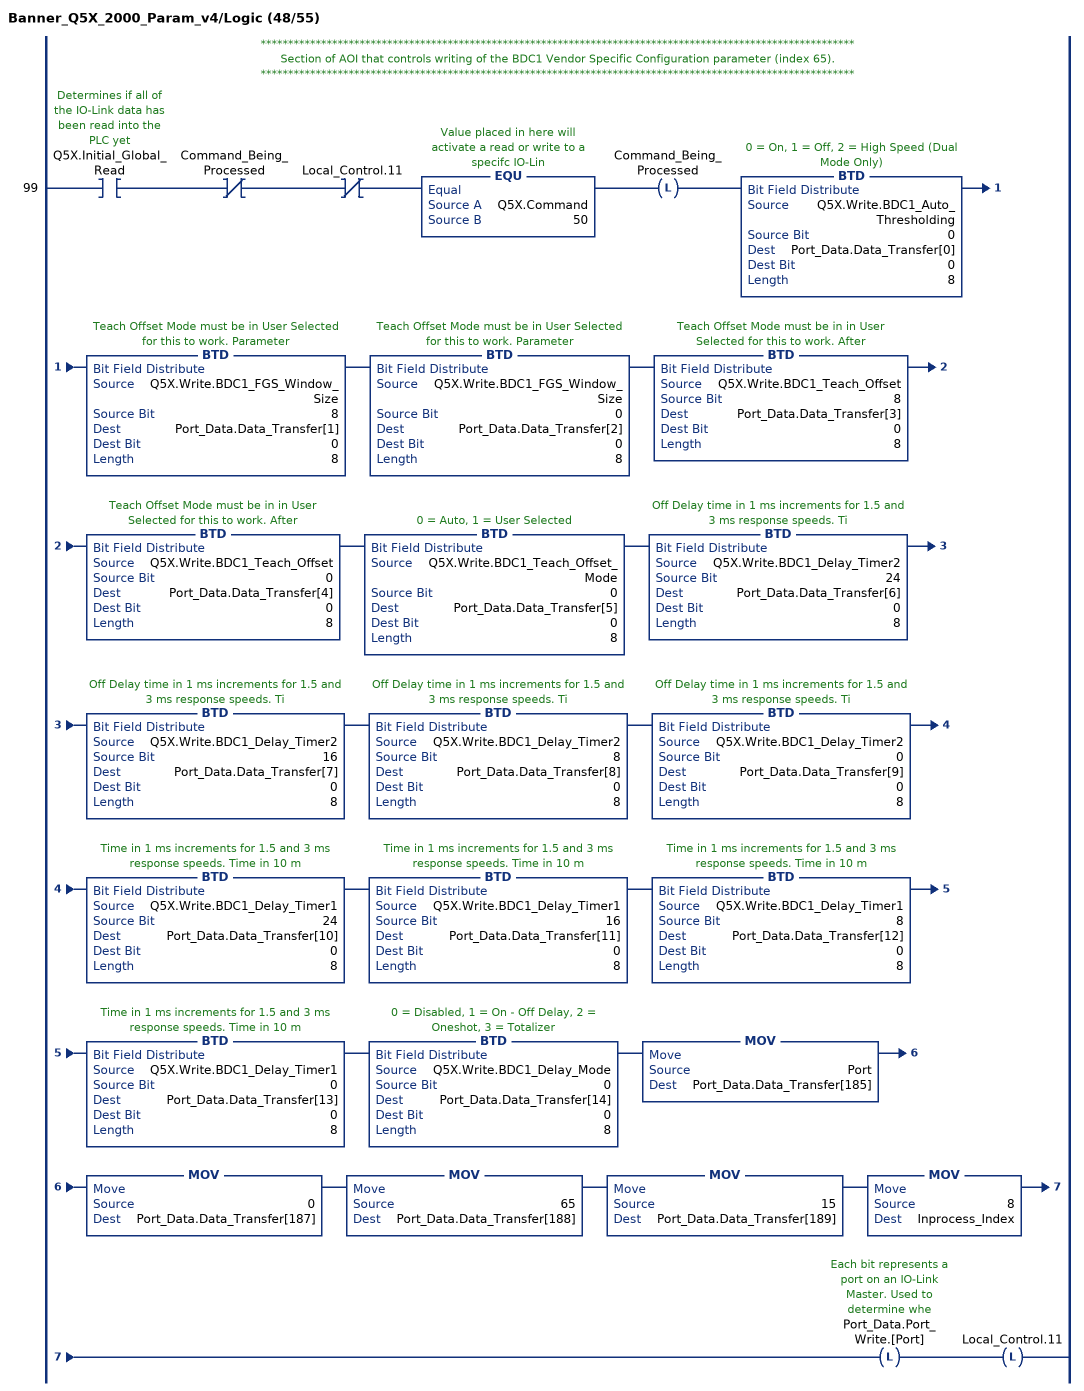
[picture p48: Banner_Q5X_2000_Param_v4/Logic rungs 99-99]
   // ************************************************************************************************************
   // Section of AOI that controls writing of the BDC1 Vendor Specific Configuration parameter (index 65).
   // ************************************************************************************************************
   99: XIC(Q5X.Initial_Global_Read)XIO(Command_Being_Processed)XIO(Local_Control.11)EQU(Q5X.Command,50)OTL(Command_Being_Processed)BTD(Q5X.Write.BDC1_Auto_Thresholding,0,Port_Data.Data_Transfer[0],0,8)BTD(Q5X.Write.BDC1_FGS_Window_Size,8,Port_Data.Data_Transfer[1],0,8)BTD(Q5X.Write.BDC1_FGS_Window_Size,0,Port_Data.Data_Transfer[2],0,8)BTD(Q5X.Write.BDC1_Teach_Offset,8,Port_Data.Data_Transfer[3],0,8)BTD(Q5X.Write.BDC1_Teach_Offset,0,Port_Data.Data_Transfer[4],0,8)BTD(Q5X.Write.BDC1_Teach_Offset_Mode,0,Port_Data.Data_Transfer[5],0,8)BTD(Q5X.Write.BDC1_Delay_Timer2,24,Port_Data.Data_Transfer[6],0,8)BTD(Q5X.Write.BDC1_Delay_Timer2,16,Port_Data.Data_Transfer[7],0,8)BTD(Q5X.Write.BDC1_Delay_Timer2,8,Port_Data.Data_Transfer[8],0,8)BTD(Q5X.Write.BDC1_Delay_Timer2,0,Port_Data.Data_Transfer[9],0,8)BTD(Q5X.Write.BDC1_Delay_Timer1,24,Port_Data.Data_Transfer[10],0,8)BTD(Q5X.Write.BDC1_Delay_Timer1,16,Port_Data.Data_Transfer[11],0,8)BTD(Q5X.Write.BDC1_Delay_Timer1,8,Port_Data.Data_Transfer[12],0,8)BTD(Q5X.Write.BDC1_Delay_Timer1,0,Port_Data.Data_Transfer[13],0,8)BTD(Q5X.Write.BDC1_Delay_Mode,0,Port_Data.Data_Transfer[14],0,8)MOV(Port,Port_Data.Data_Transfer[185])MOV(0,Port_Data.Data_Transfer[187])MOV(65,Port_Data.Data_Transfer[188])MOV(15,Port_Data.Data_Transfer[189])MOV(8,Inprocess_Index)OTL(Port_Data.Port_Write.[Port])OTL(Local_Control.11);
